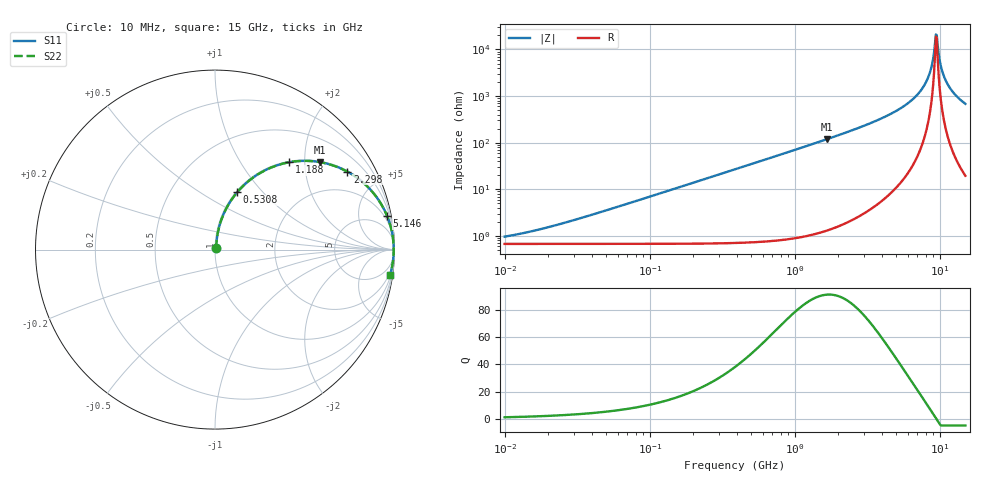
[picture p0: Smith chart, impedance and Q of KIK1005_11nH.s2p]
!version-3
!date-01.2023
!Series
# Hz S RI R 50
!Freq ReS11 ImS11 ReS21 ImS21 ReS12 ImS12 ReS22 ImS22
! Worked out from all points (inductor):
!   500 points, 10 MHz to 15 GHz, reference 50 ohm
!   read as one part in series: L = 11 nH near 29.58 MHz
!   highest Q = 91.4 at 1.665 GHz (marker M1), where L = 11.4 nH
!   self-resonance near 9.385 GHz
!   S11 on the Smith chart (normalised r, x): 10 MHz: 1.01, +0.01; 530.8 MHz: 1.01, +0.74; 1.188 GHz: 1.02, +1.67; 2.298 GHz: 1.04, +3.38; 5.146 GHz: 1, +10; 15 GHz: 1, -14
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1e7  0.00673 0.00682  0.9933 -0.00682  0.9933 -0.00682  0.00673 0.00682
3.424937e7  0.00723 0.0233  0.9928 -0.0233  0.9928 -0.0233  0.00723 0.0233
1.155953e8  0.0129 0.0783  0.9871 -0.0783  0.9871 -0.0783  0.0129 0.0783
3.901468e8  0.0736 0.2485  0.9264 -0.2485  0.9264 -0.2485  0.0736 0.2485
5.307515e8  0.1241 0.3199  0.8759 -0.3199  0.8759 -0.3199  0.1241 0.3199
1.188397e9  0.4116 0.4863  0.5884 -0.4863  0.5884 -0.4863  0.4116 0.4863
1.316788e9  0.4632 0.493  0.5368 -0.493  0.5368 -0.493  0.4632 0.493
1.664771e9  0.5842 0.4874  0.4158 -0.4874  0.4158 -0.4874  0.5842 0.4874
2.298172e9  0.7379 0.4341  0.2621 -0.4341  0.2621 -0.4341  0.7379 0.4341
4.444302e9  0.9356 0.2361  0.0644 -0.2361  0.0644 -0.2361  0.9356 0.2361
5.145797e9  0.9582 0.1886  0.0418 -0.1886  0.0418 -0.1886  0.9582 0.1886
6.601706e9  0.9833 0.1098  0.0167 -0.1098  0.0167 -0.1098  0.9833 0.1098
7.871094e9  0.9925 0.0556  0.00745 -0.0556  0.00745 -0.0556  0.9925 0.0556
8.594579e9  0.9949 0.0288  0.00514 -0.0288  0.00514 -0.0288  0.9949 0.0288
8.850227e9  0.9953 0.0199  0.00469 -0.0199  0.00469 -0.0199  0.9953 0.0199
9.248028e9  0.9957 0.00651  0.00432 -0.00651  0.00432 -0.00651  0.9957 0.00651
9.384563e9  0.9957 0.00206  0.00428 -0.00206  0.00428 -0.00206  0.9957 0.00206
9.66371e9  0.9957 -0.00685  0.00431 0.00685  0.00431 0.00685  0.9957 -0.00685
1.024716e10  0.9951 -0.0247  0.00486 0.0247  0.00486 0.0247  0.9951 -0.0247
1.102626e10  0.9935 -0.047  0.00645 0.047  0.00645 0.047  0.9935 -0.047
1.258092e10  0.9881 -0.0875  0.0119 0.0875  0.0119 0.0875  0.9881 -0.0875
1.5e10  0.975 -0.1424  0.025 0.1424  0.025 0.1424  0.975 -0.1424
